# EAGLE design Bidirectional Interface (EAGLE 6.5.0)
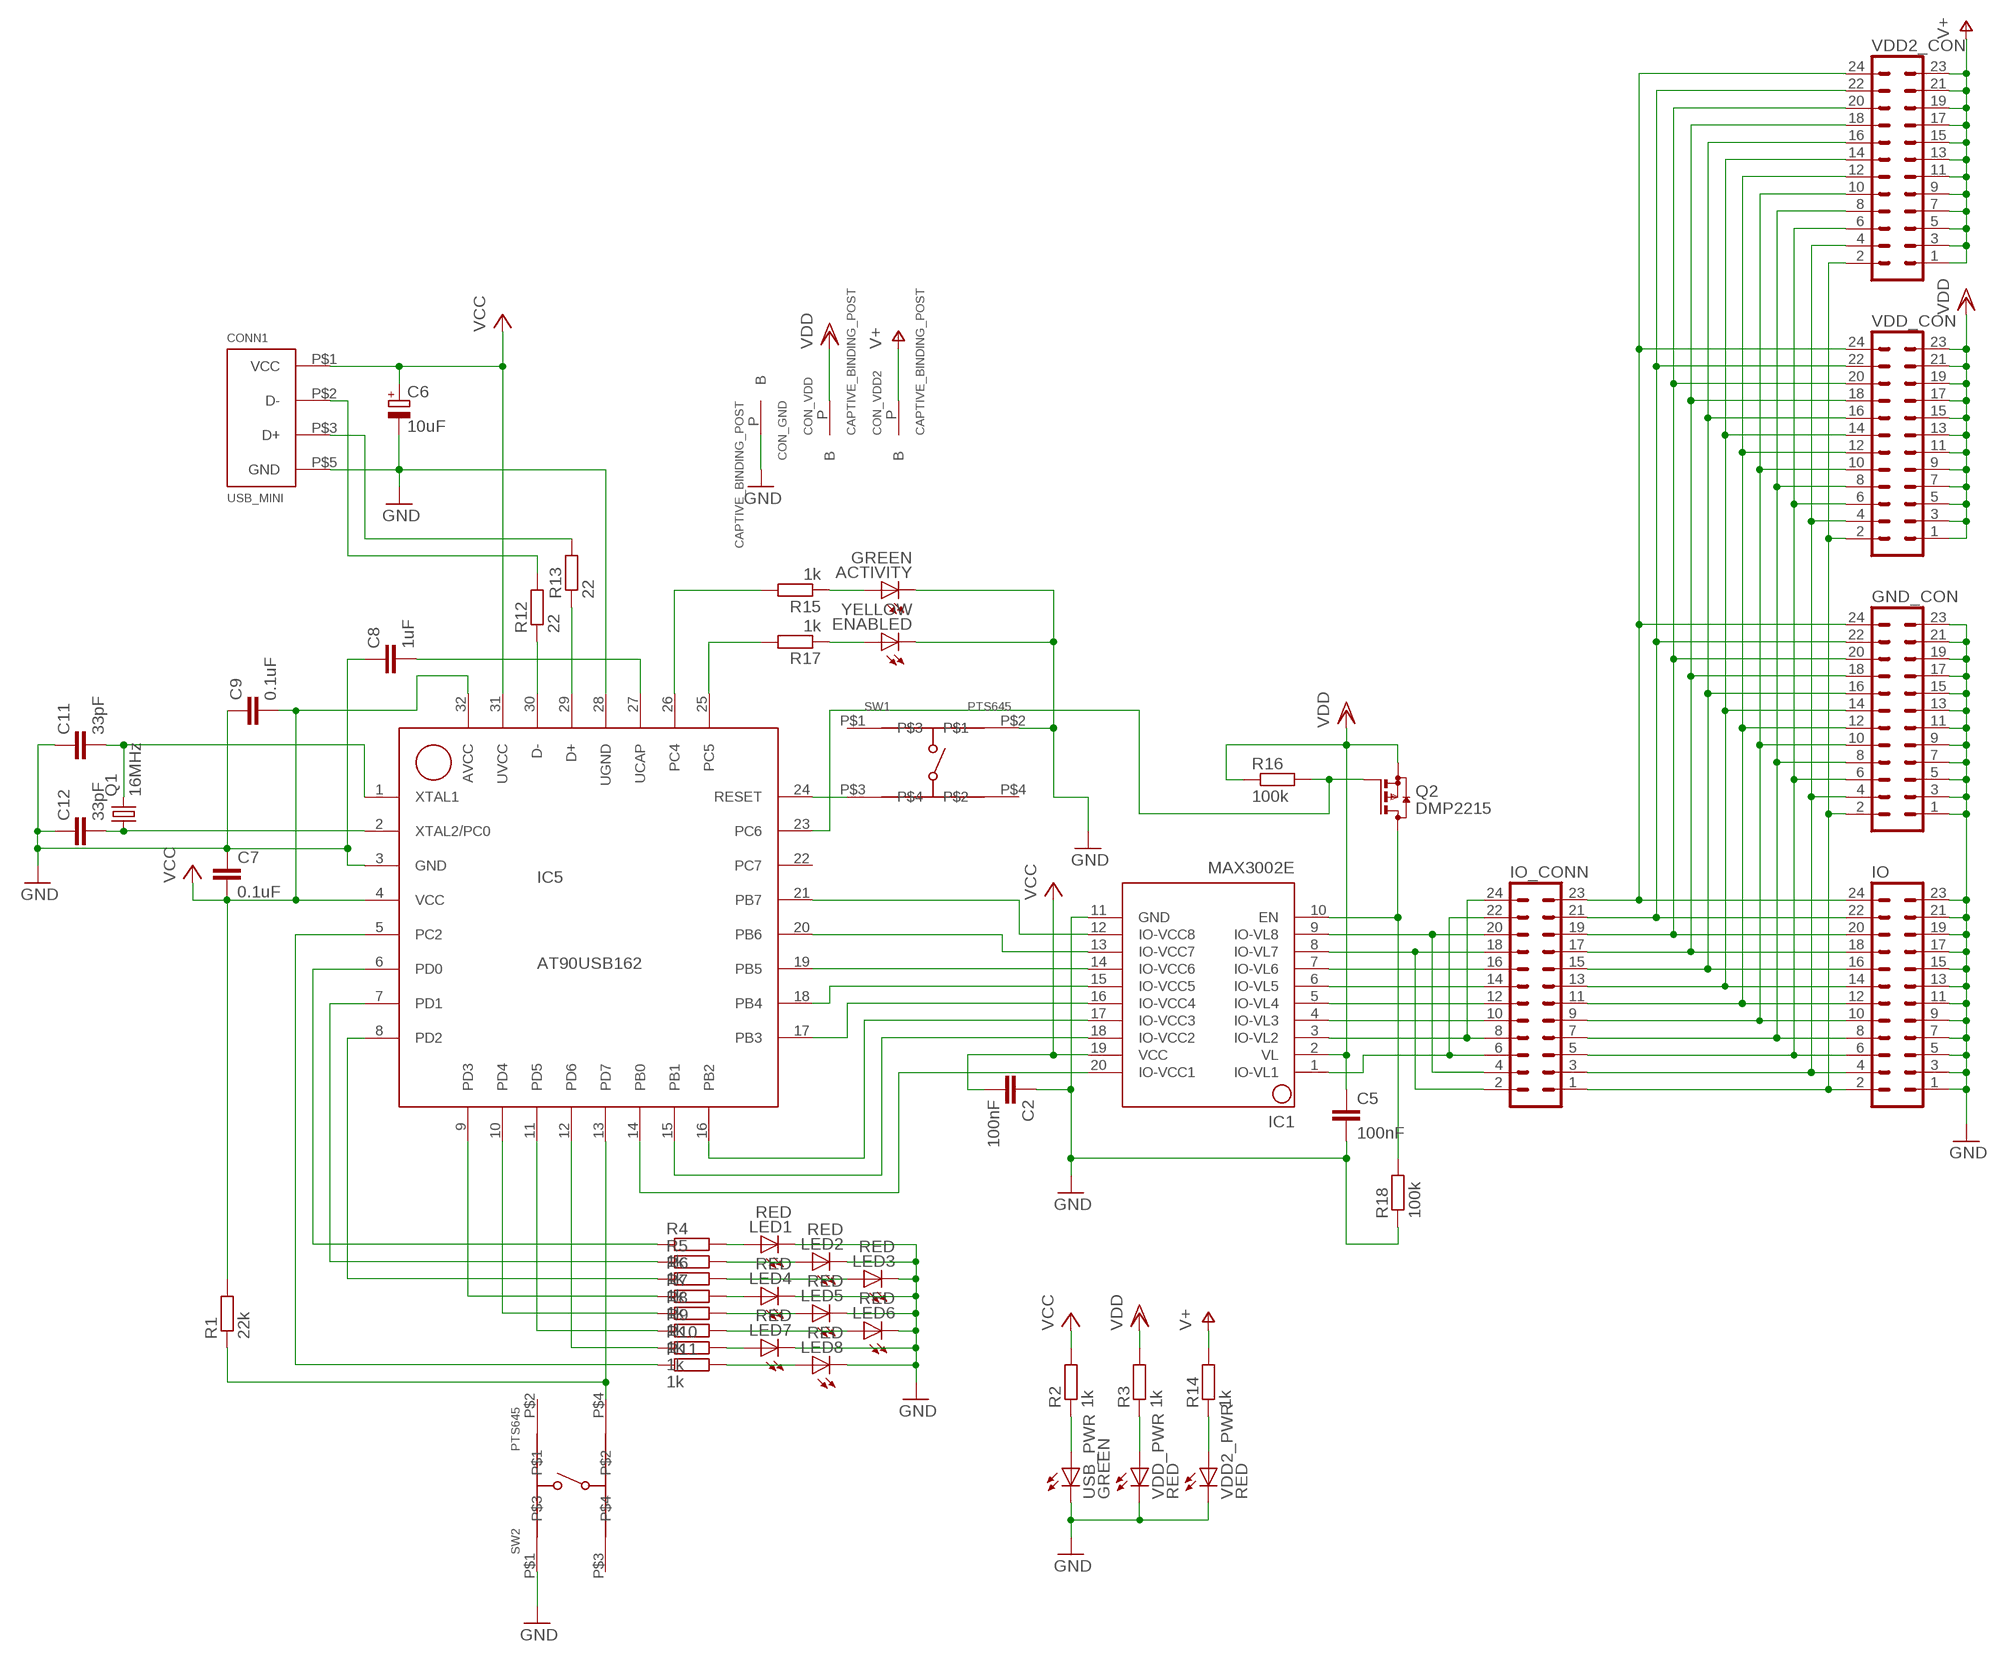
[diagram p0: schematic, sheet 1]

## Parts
ACTIVITY  GREEN  LEDCHIPLED_0805  [CHIPLED_0805]
C2  100nF  C-EUC0603  [C0603]
C5  100nF  C-EUC0603  [C0603]
C6  10uF  CPOL-EUSMCA  [SMC_A]
C7  0.1uF  C-EUC0603  [C0603]
C8  1uF  C-EUC0603  [C0603]
C9  0.1uF  C-EUC0603  [C0603]
C11  33pF  C-EUC0603  [C0603]
C12  33pF  C-EUC0603  [C0603]
CON_GND  CAPTIVE_BINDING_POST  [CAPTIVE_BINDING_POST]
CON_VDD  CAPTIVE_BINDING_POST  [CAPTIVE_BINDING_POST]
CON_VDD2  CAPTIVE_BINDING_POST  [CAPTIVE_BINDING_POST]
CONN1  USB_MINI  [SMD_MINI_USB]
ENABLED  YELLOW  LEDCHIPLED_0805  [CHIPLED_0805]
GND_CON  MA12-2  [MA12-2]
IC1  MAX3002E  [TSSOP20]
IC5  AT90USB162  [TQFP32-08]
IO  MA12-2  [MA12-2]
IO_CONN  MA12-2  [MA12-2]
LED1  RED  LEDCHIPLED_0805  [CHIPLED_0805]
LED2  RED  LEDCHIPLED_0805  [CHIPLED_0805]
LED3  RED  LEDCHIPLED_0805  [CHIPLED_0805]
LED4  RED  LEDCHIPLED_0805  [CHIPLED_0805]
LED5  RED  LEDCHIPLED_0805  [CHIPLED_0805]
LED6  RED  LEDCHIPLED_0805  [CHIPLED_0805]
LED7  RED  LEDCHIPLED_0805  [CHIPLED_0805]
LED8  RED  LEDCHIPLED_0805  [CHIPLED_0805]
Q1  16MHz  NX8045GB  [NX8045]
Q2  DMP2215  BSS84  [SOT23]
R1  22k  R-EU_R0603  [R0603]
R2  1k  R-EU_R0603  [R0603]
R3  1k  R-EU_R0603  [R0603]
R4  1k  R-EU_R0603  [R0603]
R5  1k  R-EU_R0603  [R0603]
R6  1k  R-EU_R0603  [R0603]
R7  1k  R-EU_R0603  [R0603]
R8  1k  R-EU_R0603  [R0603]
R9  1k  R-EU_R0603  [R0603]
R10  1k  R-EU_R0603  [R0603]
R11  1k  R-EU_R0603  [R0603]
R12  22  R-EU_R0603  [R0603]
R13  22  R-EU_R0603  [R0603]
R14  1k  R-EU_R0603  [R0603]
R15  1k  R-EU_R0603  [R0603]
R16  100k  R-EU_R0603  [R0603]
R17  1k  R-EU_R0603  [R0603]
R18  100k  R-EU_R0603  [R0603]
SW1  PTS645  [PTS645]
SW2  PTS645  [PTS645]
USB_PWR  GREEN  LEDCHIPLED_0805  [CHIPLED_0805]
VDD2_CON  MA12-2  [MA12-2]
VDD2_PWR  RED  LEDCHIPLED_1206  [CHIPLED_1206]
VDD_CON  MA12-2  [MA12-2]
VDD_PWR  RED  LEDCHIPLED_1206  [CHIPLED_1206]

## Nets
GND: ACTIVITY.C C2.1 C5.2 C6.- C7.1 C8.1 C9.1 C11.1 C12.1 CON_GND.P(B) CONN1.P$5(GND) ENABLED.C GND_CON.1 GND_CON.3 GND_CON.5 GND_CON.7 GND_CON.9 GND_CON.11 GND_CON.13 GND_CON.15 GND_CON.17 GND_CON.19 GND_CON.21 GND_CON.23 IC1.11(GND) IC5.3(GND) IC5.28(UGND) IO.1 IO.3 IO.5 IO.7 IO.9 IO.11 IO.13 IO.15 IO.17 IO.19 IO.21 IO.23 LED1.C LED2.C LED3.C LED4.C LED5.C LED6.C LED7.C LED8.C R18.1 SW1.P$2 SW2.P$1 USB_PWR.C VDD2_PWR.C VDD_PWR.C
N$1: CONN1.P$3(D+) R13.2
N$2: CONN1.P$2(D-) R12.2
N$3: IC5.13(PD7) R1.1 SW2.P$4
N$4: IC1.20(IO-VCC1) IC5.14(PB0)
N$5: IC1.18(IO-VCC2) IC5.15(PB1)
N$6: IC1.17(IO-VCC3) IC5.16(PB2)
N$7: IC1.16(IO-VCC4) IC5.17(PB3)
N$8: IC1.15(IO-VCC5) IC5.18(PB4)
N$9: IC1.14(IO-VCC6) IC5.19(PB5)
N$10: IC1.13(IO-VCC7) IC5.20(PB6)
N$11: IC1.12(IO-VCC8) IC5.21(PB7)
N$12: IC1.9(IO-VL8) IO_CONN.4 IO_CONN.20
N$13: IC5.26(PC4) R15.2
N$14: IC5.24(RESET) SW1.P$3
N$15: R2.1 USB_PWR.A
N$16: R3.1 VDD_PWR.A
N$17: IC1.8(IO-VL7) IO_CONN.2 IO_CONN.18
N$18: IC1.7(IO-VL6) IO_CONN.16
N$19: R14.1 VDD2_PWR.A
N$20: IC1.6(IO-VL5) IO_CONN.14
N$21: ACTIVITY.A R15.1
N$22: IC1.5(IO-VL4) IO_CONN.12
N$23: IC1.4(IO-VL3) IO_CONN.10
N$24: IC1.3(IO-VL2) IO_CONN.8 IO_CONN.24
N$25: IC1.1(IO-VL1) IO_CONN.6 IO_CONN.22
N$26: GND_CON.24 IO.24 IO_CONN.23 VDD2_CON.24 VDD_CON.24
N$27: GND_CON.22 IO.22 IO_CONN.21 VDD2_CON.22 VDD_CON.22
N$28: GND_CON.20 IO.20 IO_CONN.19 VDD2_CON.20 VDD_CON.20
N$29: GND_CON.18 IO.18 IO_CONN.17 VDD2_CON.18 VDD_CON.18
N$30: GND_CON.16 IO.16 IO_CONN.15 VDD2_CON.16 VDD_CON.16
N$31: GND_CON.14 IO.14 IO_CONN.13 VDD2_CON.14 VDD_CON.14
N$32: GND_CON.12 IO.12 IO_CONN.11 VDD2_CON.12 VDD_CON.12
N$33: GND_CON.10 IO.10 IO_CONN.9 VDD2_CON.10 VDD_CON.10
N$34: GND_CON.8 IO.8 IO_CONN.7 VDD2_CON.8 VDD_CON.8
N$35: GND_CON.6 IO.6 IO_CONN.5 VDD2_CON.6 VDD_CON.6
N$36: GND_CON.4 IO.4 IO_CONN.3 VDD2_CON.4 VDD_CON.4
N$37: GND_CON.2 IO.2 IO_CONN.1 VDD2_CON.2 VDD_CON.2
N$38: IC5.25(PC5) R17.2
N$39: IC5.6(PD0) R4.1
N$40: IC5.7(PD1) R5.1
N$41: IC5.8(PD2) R6.1
N$42: IC5.9(PD3) R7.1
N$43: IC5.10(PD4) R8.1
N$44: IC5.11(PD5) R9.1
N$45: IC5.12(PD6) R10.1
N$46: IC5.5(PC2) R11.1
N$47: LED1.A R4.2
N$48: LED2.A R5.2
N$49: LED3.A R6.2
N$50: LED4.A R7.2
N$51: LED5.A R8.2
N$52: LED6.A R9.2
N$53: LED7.A R10.2
N$54: LED8.A R11.2
N$55: IC1.10(EN) Q2.3(D) R18.2
N$56: IC5.23(PC6) Q2.1(G) R16.2
N$57: ENABLED.A R17.1
N$59: C8.2 IC5.27(UCAP)
N$69: IC5.30(D-) R12.1
N$70: IC5.29(D+) R13.1
N$73: C12.2 IC5.2(XTAL2/PC0) Q1.P$1
N$74: C11.2 IC5.1(XTAL1) Q1.P$2
V+: CON_VDD2.P(B) R14.2 VDD2_CON.1 VDD2_CON.3 VDD2_CON.5 VDD2_CON.7 VDD2_CON.9 VDD2_CON.11 VDD2_CON.13 VDD2_CON.15 VDD2_CON.17 VDD2_CON.19 VDD2_CON.21 VDD2_CON.23
VCC: C2.2 C6.+ C7.2 C9.2 CONN1.P$1(VCC) IC1.19(VCC) IC5.4(VCC) IC5.31(UVCC) IC5.32(AVCC) R1.2 R2.2
VDD: C5.1 CON_VDD.P(B) IC1.2(VL) Q2.2(S) R3.2 R16.1 VDD_CON.1 VDD_CON.3 VDD_CON.5 VDD_CON.7 VDD_CON.9 VDD_CON.11 VDD_CON.13 VDD_CON.15 VDD_CON.17 VDD_CON.19 VDD_CON.21 VDD_CON.23
Unconnected: IC5.22(PC7) SW1.P$1 SW1.P$4 SW2.P$2 SW2.P$3

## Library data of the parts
ACTIVITY ENABLED LED1-LED8 USB_PWR VDD2_PWR VDD_PWR = led:LED: LED
C2 C5 C7-C9 C11 C12 = rcl:C-EU: CAPACITOR, European symbol
C6 = rcl:CPOL-EU: POLARIZED CAPACITOR, European symbol
CON_GND CON_VDD CON_VDD2 = nicholas:CAPTIVE_BINDING_POST
CONN1 = nicholas:USB_MINI
GND_CON IO IO_CONN VDD2_CON VDD_CON = nicholas:MA12-2: PIN HEADER
IC1 = nicholas:MAX3002
IC5 = nicholas:AT90USB
Q1 = nicholas:NX8045GB
Q2 = transistor-small-signal:BSS84: P-CHANNEL MOS FET
R1-R18 = rcl:R-EU_: RESISTOR, European symbol
SW1 SW2 = nicholas:PTS645

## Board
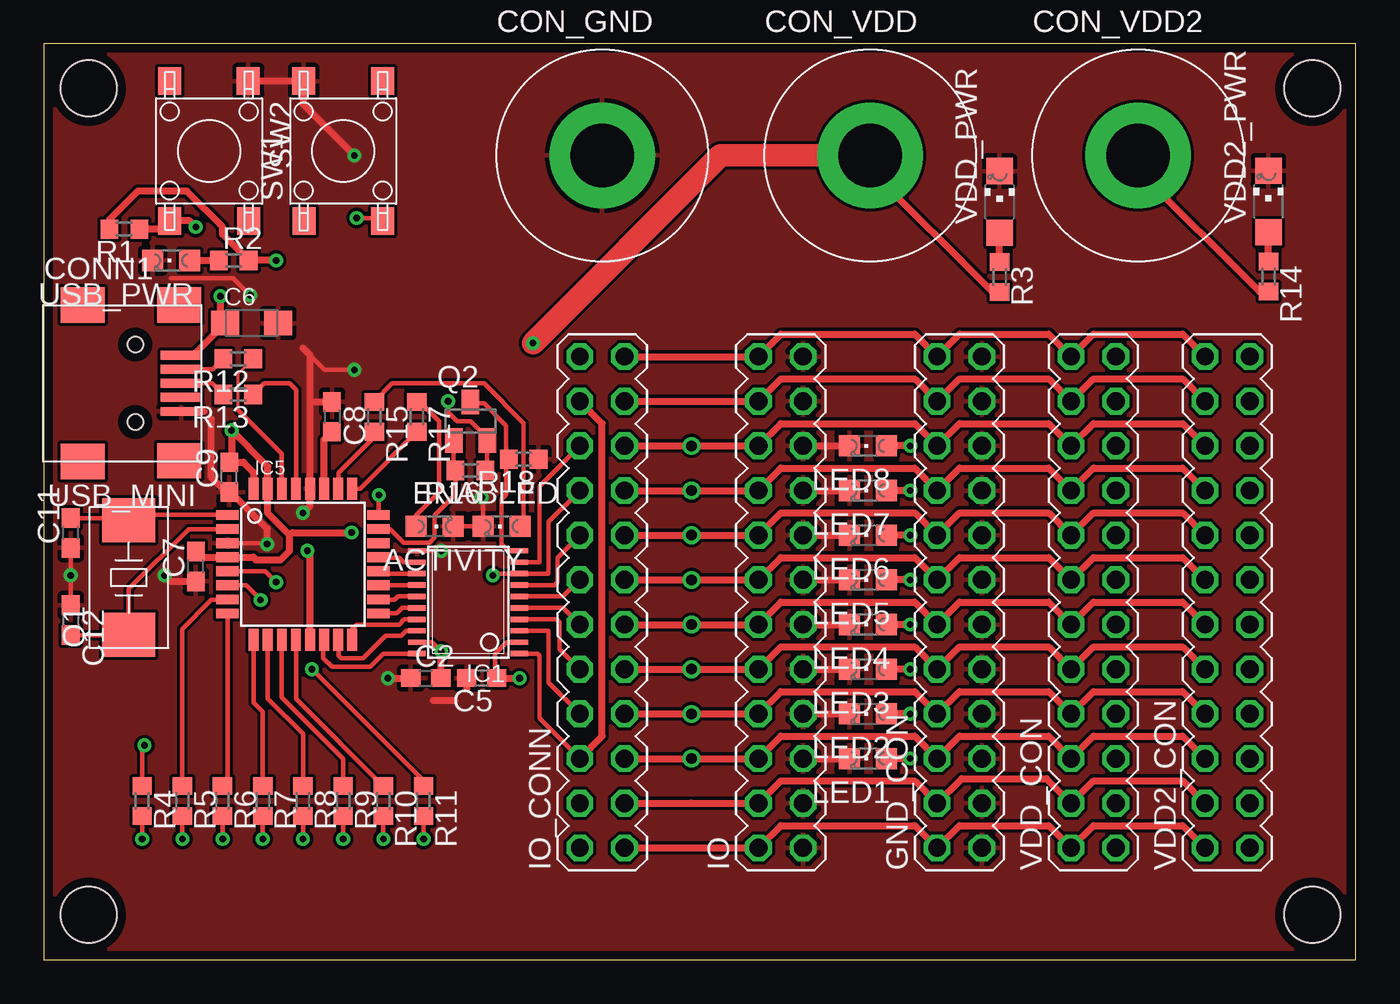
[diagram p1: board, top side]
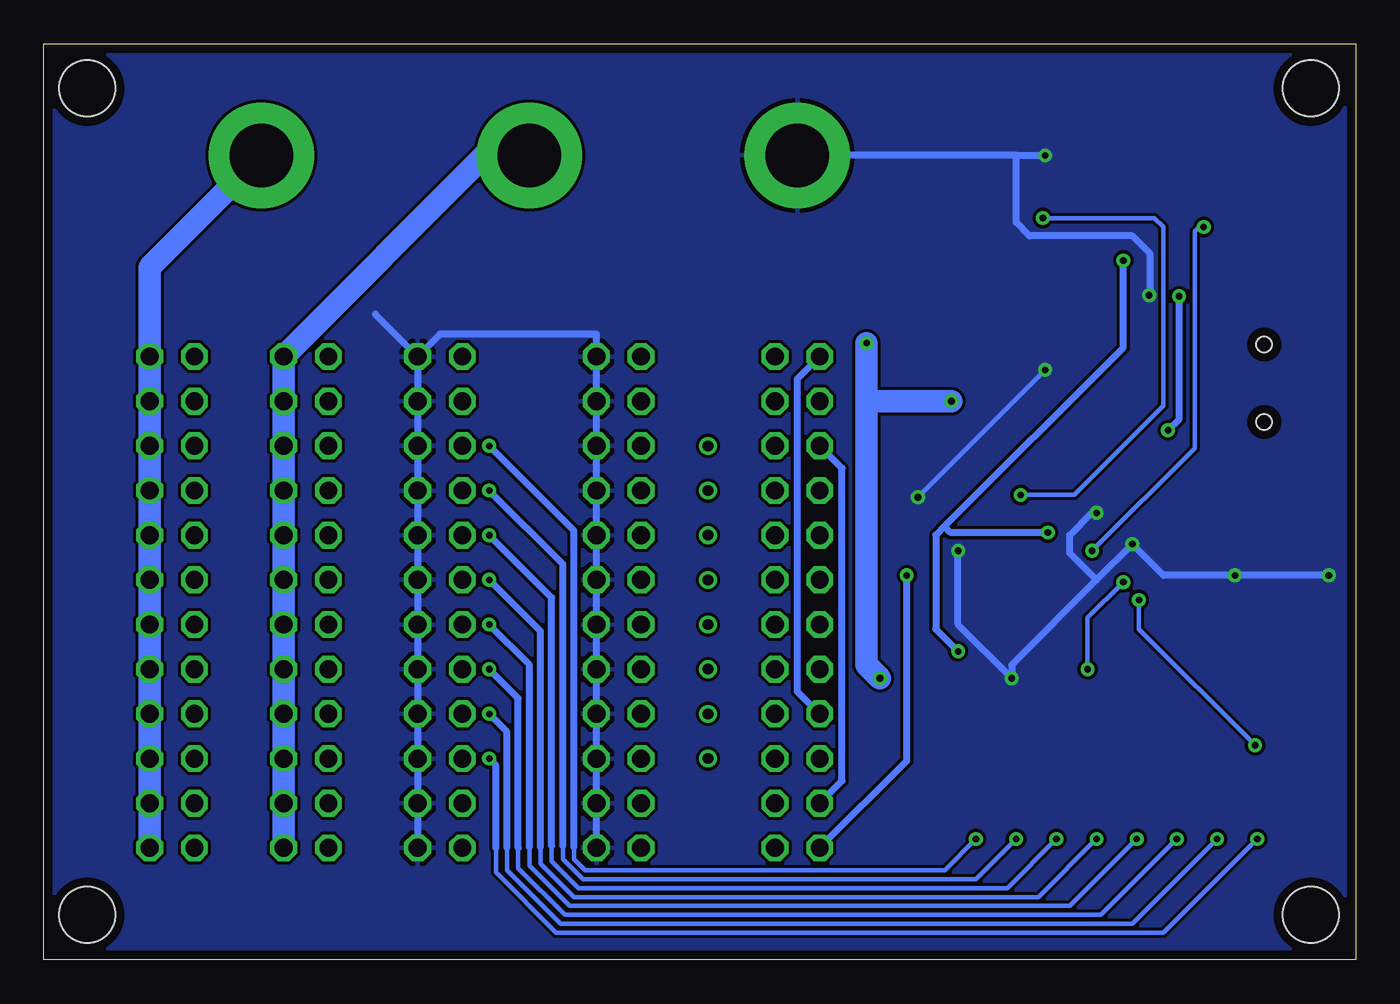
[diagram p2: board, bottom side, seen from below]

Size 74.6 x 52.06 mm. Coordinates in mm from the lower left corner, seen from the top.
Outline: 0,0 74.6,0 74.6,52.06 0,52.06 0,0
Copper layers (1*16): Top 0.035mm / dielectric 1.5mm / Bottom 0.035mm
Design rules "GoldPhoenix *": minimum track width 7mil, minimum drill 15mil, track to track 7mil, track to pad 7mil, pad to pad 7mil, via to via 7mil, smd to smd 7mil, copper to edge 20mil, drill to drill 8mil, minimum pad ring 10mil, minimum via ring 8mil, stop-mask expansion 4mil, vias tented up to drill 15mil, thermal gap 10mil
Holes 3.2 mm at 2.54,2.54 72.14,2.54 72.14,49.53 2.54,49.53

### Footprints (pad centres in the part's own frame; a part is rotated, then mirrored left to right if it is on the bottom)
CHIPLED_0805 = smd 1.2 x 1.2: A 0,-1.05; C 0,1.05
C0603 = smd 1.1 x 1: 1 -0.85,0; 2 0.85,0
SMC_A = smd 1.6 x 1.4: + -1.5,0; - 1.5,0
CAPTIVE_BINDING_POST = drill 3.6 pad 6: P 0,0
SMD_MINI_USB = smd 2.5 x 2: L1 -2.25,4.45; L2 3.25,4.45; L3 3.25,-4.4; L4 -2.25,-4.45 | smd 2.3 x 0.5: P$1 3.35,1.6; P$2 3.35,0.8; P$3 3.35,0; P$4 3.35,-0.8; P$5 3.35,-1.6 | hole 0.9: 0.75,2.2; 0.75,-2.2
MA12-2 = drill 1.016 octagon: 1 -13.97,-1.27; 2 -13.97,1.27; 3 -11.43,-1.27; 4 -11.43,1.27; 5 -8.89,-1.27; 6 -8.89,1.27; 7 -6.35,-1.27; 8 -6.35,1.27; 9 -3.81,-1.27; 10 -3.81,1.27; 11 -1.27,-1.27; 12 -1.27,1.27; 13 1.27,-1.27; 14 1.27,1.27; 15 3.81,-1.27; 16 3.81,1.27; 17 6.35,-1.27; 18 6.35,1.27; 19 8.89,-1.27; 20 8.89,1.27; 21 11.43,-1.27; 22 11.43,1.27; 23 13.97,-1.27; 24 13.97,1.27
TSSOP20 = smd 0.305 x 0.991: 1 -2.925,-2.918; 2 -2.275,-2.918; 3 -1.625,-2.918; 4 -0.975,-2.918; 5 -0.325,-2.918; 6 0.325,-2.918; 7 0.975,-2.918; 8 1.625,-2.918; 9 2.275,-2.918; 10 2.925,-2.918; 11 2.925,2.918; 12 2.275,2.918; 13 1.625,2.918; 14 0.975,2.918; 15 0.325,2.918; 16 -0.325,2.918; 17 -0.975,2.918; 18 -1.625,2.918; 19 -2.275,2.918; 20 -2.925,2.918
TQFP32-08 = smd 1.27 x 0.559: 1 -4.293,2.8; 2 -4.293,2; 3 -4.293,1.2; 4 -4.293,0.4; 5 -4.293,-0.4; 6 -4.293,-1.2; 7 -4.293,-2; 8 -4.293,-2.8; 17 4.293,-2.8; 18 4.293,-2; 19 4.293,-1.2; 20 4.293,-0.4; 21 4.293,0.4; 22 4.293,1.2; 23 4.293,2; 24 4.293,2.8 | smd 0.559 x 1.27: 9 -2.8,-4.293; 10 -2,-4.293; 11 -1.2,-4.293; 12 -0.4,-4.293; 13 0.4,-4.293; 14 1.2,-4.293; 15 2,-4.293; 16 2.8,-4.293; 25 2.8,4.293; 26 2,4.293; 27 1.2,4.293; 28 0.4,4.293; 29 -0.4,4.293; 30 -1.2,4.293; 31 -2,4.293; 32 -2.8,4.293
NX8045 = smd 2.5 x 3: P$1 -3.25,0; P$2 3.25,0
SOT23 = smd 1 x 1.4: 1 -0.95,-1.1; 2 0.95,-1.1; 3 0,1.1
R0603 = smd 1 x 1.1: 1 -0.85,0; 2 0.85,0
PTS645 = smd 1.55 x 1.3: P$1 -3.975,2.225; P$2 3.975,2.25; P$3 -3.975,-2.25; P$4 3.975,-2.25
CHIPLED_1206 = smd 1.5 x 1.5: A 0,-1.75; C 0,1.75

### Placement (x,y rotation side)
ACTIVITY  26.04,24.64 90 top
C2  21.72,16 0 top
C5  24.89,16 180 top
C6  11.81,36.2 0 top
C7  8.64,22.35 90 top
C8  16.38,30.86 270 top
C9  10.54,27.43 90 top
C11  1.52,24.26 90 top
C12  1.52,19.3 270 top
CON_GND  31.75,45.72 0 top
CON_VDD  46.99,45.72 0 top
CON_VDD2  62.23,45.72 0 top
CONN1  4.45,32.77 0 top
ENABLED  22.23,24.64 270 top
GND_CON  52.07,20.32 90 top
IC1  24.13,20.32 90 top
IC5  14.73,22.48 0 top
IO  41.91,20.32 90 top
IO_CONN  31.75,20.32 90 top
LED1  46.86,11.43 90 top
LED2  46.86,13.97 90 top
LED3  46.86,16.51 90 top
LED4  46.86,19.05 90 top
LED5  46.86,21.59 90 top
LED6  46.86,24.13 90 top
LED7  46.86,26.67 90 top
LED8  46.86,29.21 90 top
Q1  4.83,21.72 90 top
Q2  24.26,30.61 0 top
R1  4.57,41.53 180 top
R2  10.79,39.75 0 top
R3  54.36,38.81 270 top
R4  5.59,9.02 270 top
R5  7.87,9.02 270 top
R6  10.16,9.02 270 top
R7  12.45,9.02 270 top
R8  14.73,9.02 270 top
R9  17.02,9.02 270 top
R10  19.3,9.02 270 top
R11  21.59,9.02 270 top
R12  11.05,34.16 180 top
R13  11.05,32.13 180 top
R14  69.65,38.84 270 top
R15  18.8,30.86 270 top
R16  24.26,27.81 180 top
R17  21.21,30.86 270 top
R18  27.28,28.45 180 top
SW1  17.02,45.97 90 top
SW2  9.4,45.97 270 top
USB_PWR  7.24,39.75 90 top
VDD2_CON  67.31,20.32 90 top
VDD2_PWR  69.65,43.1 0 top
VDD_CON  59.69,20.32 90 top
VDD_PWR  54.36,43.08 0 top

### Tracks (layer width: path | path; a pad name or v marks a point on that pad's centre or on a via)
GND  (via drill 0.38)
  Top 0.254: C11.1 v1.52,21.84 C12.1 | v12.7,23.62 12.64,23.68 IC5.3 | IC1.11 v22.6,23.25 v22.61,23.24 | 7.21,38.73 10.77,38.73 v11.74,37.77 | ENABLED.C ACTIVITY.C 24.98,26.2 v24.89,26.29 | v17.65,33.53 15.98,33.53 14.72,34.79
  Top 0.406: IO.19 LED8.C | IO.17 LED7.C | IO.15 LED6.C | IO.13 LED5.C | IO.11 LED4.C | IO.9 LED3.C | IO.7 LED2.C | IO.5 LED1.C | CONN1.P$5 9.09,31.17 | v12.7,23.62 12.7,24.51 10.63,26.58 C9.1 10.45,26.67 10.29,26.67 9.53,27.43 9.53,30.73 | 14.72,34.79 15.13,34.37 15.13,31.5 | 15.13,31.5 IC5.28 15.13,25.8 v14.73,25.4 | v19.56,16 C2.1 | C5.2 24.04,15.41 | 22.14,14.73 23.37,14.73 | C7.1 7.2,21.5 v6.86,21.84 | C8.1 15.35,31.71 arc90 15.13,31.5 | SW2.P$1 SW1.P$2 14.77,48.6 v17.65,45.72
  Bottom 0.254: v17.65,33.53 v24.89,26.29
  Bottom 0.406: IO.1 IO.3 IO.5 IO.7 IO.9 IO.11 IO.13 IO.15 IO.17 IO.19 IO.21 IO.23 43.18,35.56 52.07,35.56 GND_CON.23 | GND_CON.1 GND_CON.3 GND_CON.5 GND_CON.7 GND_CON.9 GND_CON.11 GND_CON.13 GND_CON.15 GND_CON.17 GND_CON.19 | GND_CON.19 GND_CON.21 GND_CON.23 | v1.52,21.84 v6.86,21.84 10.92,21.84 v12.7,23.62 14.73,21.59 | 14.73,21.59 19.56,16.76 v19.56,16 22.61,19.05 v22.61,23.24 | v11.74,37.77 11.68,37.82 11.68,40.13 12.7,41.15 18.54,41.15 19.3,41.91 19.3,45.72 | GND_CON.23 55.75,36.7 | v14.73,25.4 14.99,25.4 16.26,24.13 16.26,23.11 14.73,21.59 | GND_CON.23 GND_CON.19 | 19.3,45.72 CON_GND.P | 19.3,45.72 v17.65,45.72
  pour Top: 0,52.07 0,0 74.93,0 74.93,52.07
  pour Bottom: 0,52.07 0,0 74.93,0 74.93,52.07
N$1
  Top 0.254: CONN1.P$3 9.56,32.77 R13.2
N$2
  Top 0.254: CONN1.P$2 9.6,33.57 R12.2
N$3  (via drill 0.38)
  Top 0.406: IC5.13 15.13,23.09 v14.99,23.24 | R1.1 6.68,41.53 SW2.P$4 8.29,42 v8.64,41.66
  Bottom 0.254: v14.99,23.24 9.14,29.08 9.14,41.4 8.89,41.66 v8.64,41.66
N$4
  Top 0.254: IC1.20 19.3,17.39 18.54,16.64 16.38,16.64 15.88,17.14 15.88,18.13 IC5.14
N$5
  Top 0.254: IC1.18 20.6,18.7 20.32,18.41 19.43,18.41 18.16,17.14 16.89,17.14 16.76,17.27 16.76,18.15 IC5.15
N$6
  Top 0.254: IC1.17 20.49,19.34 20.19,19.05 17.78,19.05 17.53,18.8 IC5.16
N$7
  Top 0.254: IC1.16 20.38,20 20.07,19.68 IC5.17
N$8
  Top 0.254: IC1.15 20.14,20.64 19.94,20.45 19.06,20.45 IC5.18
N$9
  Top 0.254: IC1.14 19.04,21.3 IC5.19
N$10
  Top 0.254: IC1.13 19.16,21.95 IC5.20
N$11
  Top 0.254: IC1.12 20.46,22.59 20.19,22.86 19.04,22.86 IC5.21
N$12
  Top 0.254: IC1.9 28.18,22.59 28.19,22.61 28.19,26.92 IO_CONN.20
  Bottom 0.406: IO_CONN.4 29.21,10.16 29.21,27.94 IO_CONN.20
N$13
  Top 0.254: R15.2 18.8,29.72 16.76,27.69 16.76,26.8 IC5.26
N$14  (via drill 0.38)
  Top 0.254: IC5.24 19.02,26.39 v19.05,26.42 | v17.78,42.16 19.1,42.16 SW1.P$3
  Bottom 0.254: v19.05,26.42 16,26.42 10.92,31.5 10.92,41.66 11.43,42.16 v17.78,42.16
N$15
  Top 0.406: USB_PWR.A R2.1
N$16
  Top 0.406: R3.1 VDD_PWR.A
N$17  (via drill 0.38)
  Top 0.254: IO_CONN.18 28.7,24.89 28.7,21.97 28.68,21.95 IC1.8 25.63,21.95 v25.53,21.84
  Bottom 0.406: IO_CONN.2 25.53,11.3 v25.53,21.84
N$18
  Top 0.254: IC1.7 29.04,21.3 29.21,21.46 29.21,22.86 IO_CONN.16
N$19
  Top 0.406: R14.1 VDD2_PWR.A
N$20
  Top 0.254: IC1.6 29.54,20.64 IO_CONN.14
N$21
  Top 0.254: R15.1 18.8,31.75 19.81,32.77 25.02,32.77 27.28,30.5 27.28,24.83 ACTIVITY.A 27.05,24.67
N$22
  Top 0.254: IC1.5 29.54,20 IO_CONN.12
N$23
  Top 0.254: IC1.4 29.17,19.34 29.34,19.18 29.34,17.65 IO_CONN.10
N$24
  Top 0.254: IC1.3 28.68,18.7 28.7,18.67 28.7,15.75 IO_CONN.8
  Bottom 0.406: IO_CONN.24 31.75,33.02 31.75,15.24 IO_CONN.8
N$25
  Top 0.254: IC1.1 28.07,17.39 28.19,17.27 28.19,13.72 IO_CONN.6
  Top 0.406: IO_CONN.22 31.75,30.48 31.75,12.7 IO_CONN.6
N$26
  Top 0.406: IO_CONN.23 IO.24 41.91,35.56 49.53,35.56 GND_CON.24 52.07,35.56 57.15,35.56 VDD_CON.24 59.69,35.56 64.77,35.56 VDD2_CON.24
N$27
  Top 0.406: IO_CONN.21 IO.22 41.91,33.02 49.53,33.02 GND_CON.22 52.07,33.02 57.15,33.02 VDD_CON.22 59.69,33.02 64.77,33.02 VDD2_CON.22
N$28  (via drill 0.6)
  Top 0.406: IO_CONN.19 v36.83,29.21 IO.20 41.91,30.48 49.53,30.48 GND_CON.20 52.07,30.48 57.15,30.48 VDD_CON.20 59.69,30.48 64.77,30.48 VDD2_CON.20
N$29  (via drill 0.6)
  Top 0.406: IO_CONN.17 v36.83,26.67 IO.18 41.91,27.94 49.53,27.94 GND_CON.18 52.07,27.94 57.15,27.94 VDD_CON.18 59.69,27.94 64.77,27.94 VDD2_CON.18
N$30  (via drill 0.6)
  Top 0.406: IO_CONN.15 v36.83,24.13 IO.16 41.91,25.4 49.53,25.4 GND_CON.16 52.07,25.4 57.15,25.4 VDD_CON.16 59.69,25.4 64.77,25.4 VDD2_CON.16
N$31  (via drill 0.6)
  Top 0.406: IO_CONN.13 v36.83,21.59 IO.14 41.91,22.86 49.53,22.86 GND_CON.14 52.07,22.86 57.15,22.86 VDD_CON.14 59.69,22.86 64.77,22.86 VDD2_CON.14
N$32  (via drill 0.6)
  Top 0.406: IO_CONN.11 v36.83,19.05 IO.12 41.91,20.32 49.53,20.32 GND_CON.12 52.07,20.32 57.15,20.32 VDD_CON.12 59.69,20.32 64.77,20.32 VDD2_CON.12
N$33  (via drill 0.6)
  Top 0.406: IO_CONN.9 v36.83,16.51 IO.10 41.91,17.78 49.53,17.78 GND_CON.10 52.07,17.78 57.15,17.78 VDD_CON.10 59.69,17.78 64.77,17.78 VDD2_CON.10
N$34  (via drill 0.6)
  Top 0.406: IO_CONN.7 v36.83,13.97 IO.8 41.91,15.24 49.53,15.24 GND_CON.8 52.07,15.24 57.15,15.24 VDD_CON.8 59.69,15.24 64.77,15.24 VDD2_CON.8
N$35  (via drill 0.6)
  Top 0.406: IO_CONN.5 v36.83,11.43 IO.6 41.91,12.7 49.53,12.7 GND_CON.6 52.07,12.7 57.15,12.7 VDD_CON.6 59.69,12.7 64.77,12.7 VDD2_CON.6
N$36
  Top 0.406: IO_CONN.3 36.83,8.89 IO.4 41.91,10.16 49.53,10.16 GND_CON.4 52.2,10.29 57.02,10.29 VDD_CON.4 59.69,10.16 64.77,10.16 VDD2_CON.4
N$37
  Top 0.406: IO_CONN.1 IO.2 41.91,7.62 49.53,7.62 GND_CON.2 52.07,7.62 57.15,7.62 VDD_CON.2 59.69,7.62 64.77,7.62 VDD2_CON.2
N$38
  Top 0.254: IC5.25 17.97,26.77 R17.2
N$39  (via drill 0.38)
  Top 0.254: R4.1 5.59,12.06 v5.71,12.19 | v12.32,20.45 11.49,21.28 IC5.6
  Bottom 0.254: v5.71,12.19 12.32,18.8 v12.32,20.45
N$40
  Top 0.254: R5.1 7.87,18.8 9.53,20.45 10.41,20.45 IC5.7
N$41
  Top 0.254: R6.1 10.44,10.15 IC5.8
N$42
  Top 0.254: R7.1 12.45,14.1 11.94,14.61 IC5.9
N$43
  Top 0.254: R8.1 14.73,12.83 12.73,14.83 IC5.10
N$44
  Top 0.254: R9.1 17.02,11.43 13.53,14.92 IC5.11
N$45
  Top 0.254: R10.1 14.33,14.84 IC5.12
N$46  (via drill 0.38)
  Top 0.254: v13.21,21.46 12.59,22.08 IC5.5 | R11.1 21.59,10.16 v15.24,16.51
  Bottom 0.254: v15.24,16.51 15.24,19.43 v13.21,21.46
N$47  (via drill 0.38)
  Top 0.254: v5.59,6.86 R4.2
  Top 0.406: v49.28,11.43 LED1.A
  Bottom 0.254: 48.9,6.35 48.9,4.95 45.47,1.52 10.92,1.52 v5.59,6.86
  Bottom 0.406: v49.28,11.43 48.9,11.05 48.9,6.35
N$48  (via drill 0.38)
  Top 0.254: v7.87,6.86 R5.2
  Top 0.406: v49.28,13.97 LED2.A
  Bottom 0.254: 48.26,6.36 48.26,5.08 45.21,2.03 12.7,2.03 v7.87,6.86
  Bottom 0.406: v49.28,13.97 48.26,12.95 48.26,6.36
N$49  (via drill 0.38)
  Top 0.254: v10.16,6.86 R6.2
  Top 0.406: v49.28,16.51 LED3.A
  Bottom 0.254: 47.62,6.35 47.62,5.21 44.96,2.54 14.48,2.54 v10.16,6.86
  Bottom 0.406: v49.28,16.51 47.62,14.86 47.62,6.35
N$50  (via drill 0.38)
  Top 0.254: v12.45,6.86 R7.2
  Top 0.406: v49.28,19.05 LED4.A
  Bottom 0.254: 46.99,6.41 46.99,5.33 44.7,3.05 16.26,3.05 v12.45,6.86
  Bottom 0.406: v49.28,19.05 46.99,16.76 46.99,6.41
N$51  (via drill 0.38)
  Top 0.254: v14.73,6.86 R8.2
  Top 0.406: v49.28,21.59 LED5.A
  Bottom 0.254: 46.35,6.4 46.35,5.46 44.45,3.56 18.03,3.56 v14.73,6.86
  Bottom 0.406: v49.28,21.59 46.35,18.67 46.35,6.4
N$52  (via drill 0.38)
  Top 0.254: v17.02,6.86 R9.2
  Top 0.406: v49.28,24.13 LED6.A
  Bottom 0.254: 45.72,6.46 45.72,5.59 44.2,4.06 19.81,4.06 v17.02,6.86
  Bottom 0.406: v49.28,24.13 45.72,20.57 45.72,6.46
N$53  (via drill 0.38)
  Top 0.254: v19.3,6.86 R10.2
  Top 0.406: v49.28,26.67 LED7.A
  Bottom 0.254: 45.09,6.45 45.09,5.71 43.94,4.57 21.59,4.57 v19.3,6.86
  Bottom 0.406: v49.28,26.67 45.09,22.48 45.09,6.45
N$54  (via drill 0.38)
  Top 0.254: v21.59,6.86 R11.2
  Top 0.406: v49.28,29.21 LED8.A
  Bottom 0.254: 44.45,6.41 44.45,5.71 43.81,5.08 23.37,5.08 v21.59,6.86
  Bottom 0.406: v49.28,29.21 44.45,24.38 44.45,6.41
N$55
  Top 0.254: IC1.10 26.41,23.25 26.04,23.62 26.04,26.16 26.29,26.42 26.29,28.45 | 26.29,28.45 26.29,30.35 25.02,31.62 24.34,31.62 Q2.3 | 26.29,28.45 R18.2
N$56
  Top 0.254: 19.06,24.51 IC5.23 19.69,24.48 20.46,23.71 21.93,23.71 22.23,24 22.23,25.27 23.41,26.45 R16.2 23.31,27.91 Q2.1
N$57
  Top 0.254: R17.1 21.38,31.71 22.48,30.61 22.48,26.58 21.18,25.27 ENABLED.A
N$59
  Top 0.406: IC5.27 15.93,29.56 C8.2
N$69
  Top 0.178: R12.1 11.05,33.31 11.05,31.24
  Top 0.254: 11.05,31.24 13.53,28.76 IC5.30
N$70
  Top 0.254: IC5.29 14.33,32.4 13.97,32.77 12.53,32.77 R13.1
N$73
  Top 0.254: IC5.2 8.22,24.48 4.83,21.08 Q1.P$1 4.81,18.45 C12.2
N$74
  Top 0.254: IC5.1 5.14,25.28 Q1.P$2 4.69,25.11 C11.2
V+
  Top 0.406: R14.2 69.12,37.99 62.23,44.88 CON_VDD2.P
  Bottom 1.27: CON_VDD2.P 68.58,39.37 VDD2_CON.23 VDD2_CON.21 VDD2_CON.19 VDD2_CON.17 VDD2_CON.15 VDD2_CON.13 VDD2_CON.11 VDD2_CON.9 VDD2_CON.7 VDD2_CON.5 VDD2_CON.3 VDD2_CON.1
VCC  (via drill 0.38)
  Top 0.254: IC1.19 22.09,18.05 v22.61,17.53
  Top 0.406: C2.2 22.57,17.49 v22.61,17.53 | C7.2 8.96,22.88 IC5.4 11.92,22.88 12.06,22.73 13.46,22.73 13.97,23.24 13.97,24.13 | v13.21,39.75 R2.2 10.16,41.24 10.16,41.66 8.13,43.69 5.33,43.69 3.72,42.08 R1.2 | IC5.32 11.94,27.69 11.34,28.28 C9.2 10.67,28.41 v10.67,30.1 12.73,28.04 IC5.31 12.73,25.37 13.97,24.13 | CONN1.P$1 8.48,34.37 C6.+ 10.03,36.47 v10.03,37.72 | 13.97,24.13 14.12,24.28 v17.5,24.28
  Bottom 0.406: v22.61,17.53 23.88,18.8 23.88,24.13 23.38,24.62 | v10.67,30.1 10.03,30.73 v10.03,37.72 | 23.38,24.62 13.21,34.8 v13.21,39.75 | v17.5,24.28 23.04,24.28 23.38,24.62
VDD  (via drill 0.38)
  Top 0.254: IC1.2 26.3,18.05 25.65,17.4 25.65,16.09 C5.1 | R16.1 25.21,27.91 Q2.2 25.21,29.66 24.26,30.61 23.5,30.61 22.99,31.11 v22.99,31.75
  Top 0.406: C5.1 v27.05,16 | R3.2 53.94,37.96 46.99,44.91 CON_VDD.P
  Top 1.27: v27.81,35.05 38.48,45.72 CON_VDD.P
  Bottom 1.27: CON_VDD.P 49.53,45.72 VDD_CON.23 VDD_CON.21 VDD_CON.19 VDD_CON.17 VDD_CON.15 VDD_CON.13 VDD_CON.11 VDD_CON.9 VDD_CON.7 VDD_CON.5 VDD_CON.3 VDD_CON.1 | 27.81,31.75 27.81,16.76 v27.05,16 | 27.81,31.75 v27.81,35.05 | 27.81,31.75 v22.99,31.75

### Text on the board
tDocu: PGM | PWR | RESET | Silicon Chip | GND | + | VDD | VDD2 | Bidirectional | S | G | Interface | 2 | 1 | OUT | 8 | ENA | ACT | 7 | 6 | 5 | 4 | 3 | 2 | 1 | 8 | 7 | I/O ENA | I/O | GND | VDD | VDD2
